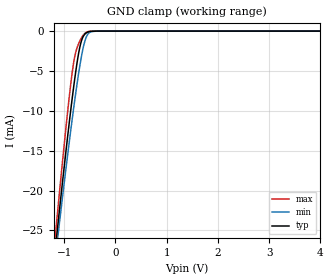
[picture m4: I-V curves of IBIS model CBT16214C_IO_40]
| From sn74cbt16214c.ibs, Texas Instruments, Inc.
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[Model]   CBT16214C_IO_40
Model_type  Terminator
| variable   typ   min   max
C_comp   8.46pF   7.26pF   11.42pF
| C_tri-state   8.46pF   7.26pF   11.42pF
[Temperature Range]   40   100   -40
| Ambient temperature   25   85   -40
[Voltage range]   4   4   4
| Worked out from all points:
|   GND clamp passes 1 mA (typ) near -0.65 V on its own axis
[GND Clamp]
| CBT16214C_IO_40
|   Voltage   I(typ)   I(min)   I(max)
-4V       -217.1mA   -203mA     -234.6mA
-1.165V   -26.95mA   -28.19mA   -25.27mA
-1.135V   -25.13mA   -26.53mA   -23.25mA
-1.105V   -23.33mA   -24.87mA   -21.25mA
-920mV    -12.63mA   -15mA      -9.476mA
-815mV    -7.098mA   -9.758mA   -4.034mA
-765mV    -4.746mA   -7.423mA   -2.48mA
-680mV    -1.666mA   -3.863mA   -1.08mA
-610mV    -508.1uA   -1.615mA   -384.4uA
-555mV    -182.6uA   -590.6uA   -116.8uA
-320mV    -1.14uA    -5.749uA   -33.8nA
4V        638.9pA    1.871nA    275.5pA
